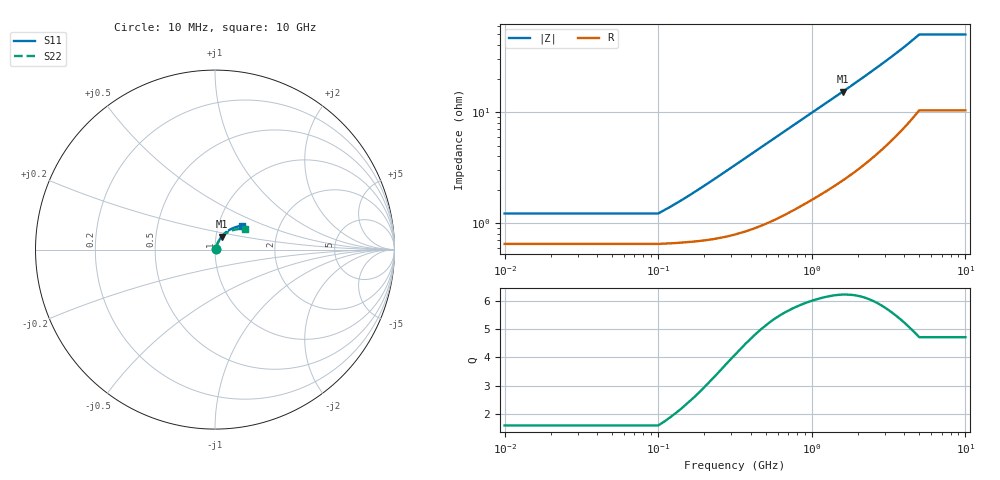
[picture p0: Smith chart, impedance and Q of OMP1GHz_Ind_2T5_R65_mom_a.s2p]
! Created Fri Jun 17 13:48:52 2016
# ghz S ma R 50
! 2 Port Network Data from SP1.SP block
! freq  magS11  angS11  magS21  angS21  magS12  angS12  magS22  angS22
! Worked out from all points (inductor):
!   1000 points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, 10 MHz to 10 GHz, reference 50 ohm
!   read as 1/Y11, port 2 shorted: L = 1.63 nH near 210 MHz
!   highest Q = 6.22 at 1.59 GHz (marker M1), where L = 1.51 nH
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0.01  0.008797 42.0  0.9935 -0.8  0.9935 -0.8  0.008802 41.9
0.06  0.008797 42.0  0.9935 -0.8  0.9935 -0.8  0.008802 41.9
0.1  0.008797 42.0  0.9935 -0.8  0.9935 -0.8  0.008802 41.9
0.14  0.01065 50.4  0.9933 -1.2  0.9933 -1.2  0.01066 50.2
0.19  0.0132 57.1  0.993 -1.6  0.993 -1.6  0.01321 56.9
0.24  0.01588 61.2  0.9926 -2.0  0.9926 -2.0  0.01589 60.9
0.34  0.02134 65.4  0.9917 -2.8  0.9917 -2.8  0.02137 65.0
0.47  0.02836 67.4  0.9901 -3.9  0.9901 -3.9  0.0284 66.8
0.62  0.03615 67.8  0.9881 -5.1  0.9881 -5.1  0.0362 67.0
0.8  0.04504 67.4  0.9854 -6.5  0.9854 -6.5  0.0451 66.3
1.02  0.05535 66.4  0.9821 -8.1  0.9821 -8.1  0.05541 65.0
1.28  0.067 65.0  0.978 -10.1  0.978 -10.1  0.06704 63.3
1.59  0.08035 63.2  0.9728 -12.3  0.9728 -12.3  0.08036 61.1
1.68  0.08414 62.6  0.9713 -13.0  0.9713 -13.0  0.08414 60.4
2.03  0.09853 60.4  0.965 -15.5  0.965 -15.5  0.09847 57.7
2.42  0.114 57.8  0.9575 -18.3  0.9575 -18.3  0.1138 54.6
3.34  0.1479 51.7  0.9383 -24.7  0.9383 -24.7  0.1473 47.3
4.14  0.1752 46.5  0.9207 -30.1  0.9207 -30.1  0.1739 41.2
5.01  0.2031 41.1  0.9012 -35.7  0.9012 -35.7  0.2009 34.9
6.67  0.2031 41.1  0.9012 -35.7  0.9012 -35.7  0.2009 34.9
8.34  0.2031 41.1  0.9012 -35.7  0.9012 -35.7  0.2009 34.9
10  0.2031 41.1  0.9012 -35.7  0.9012 -35.7  0.2009 34.9
